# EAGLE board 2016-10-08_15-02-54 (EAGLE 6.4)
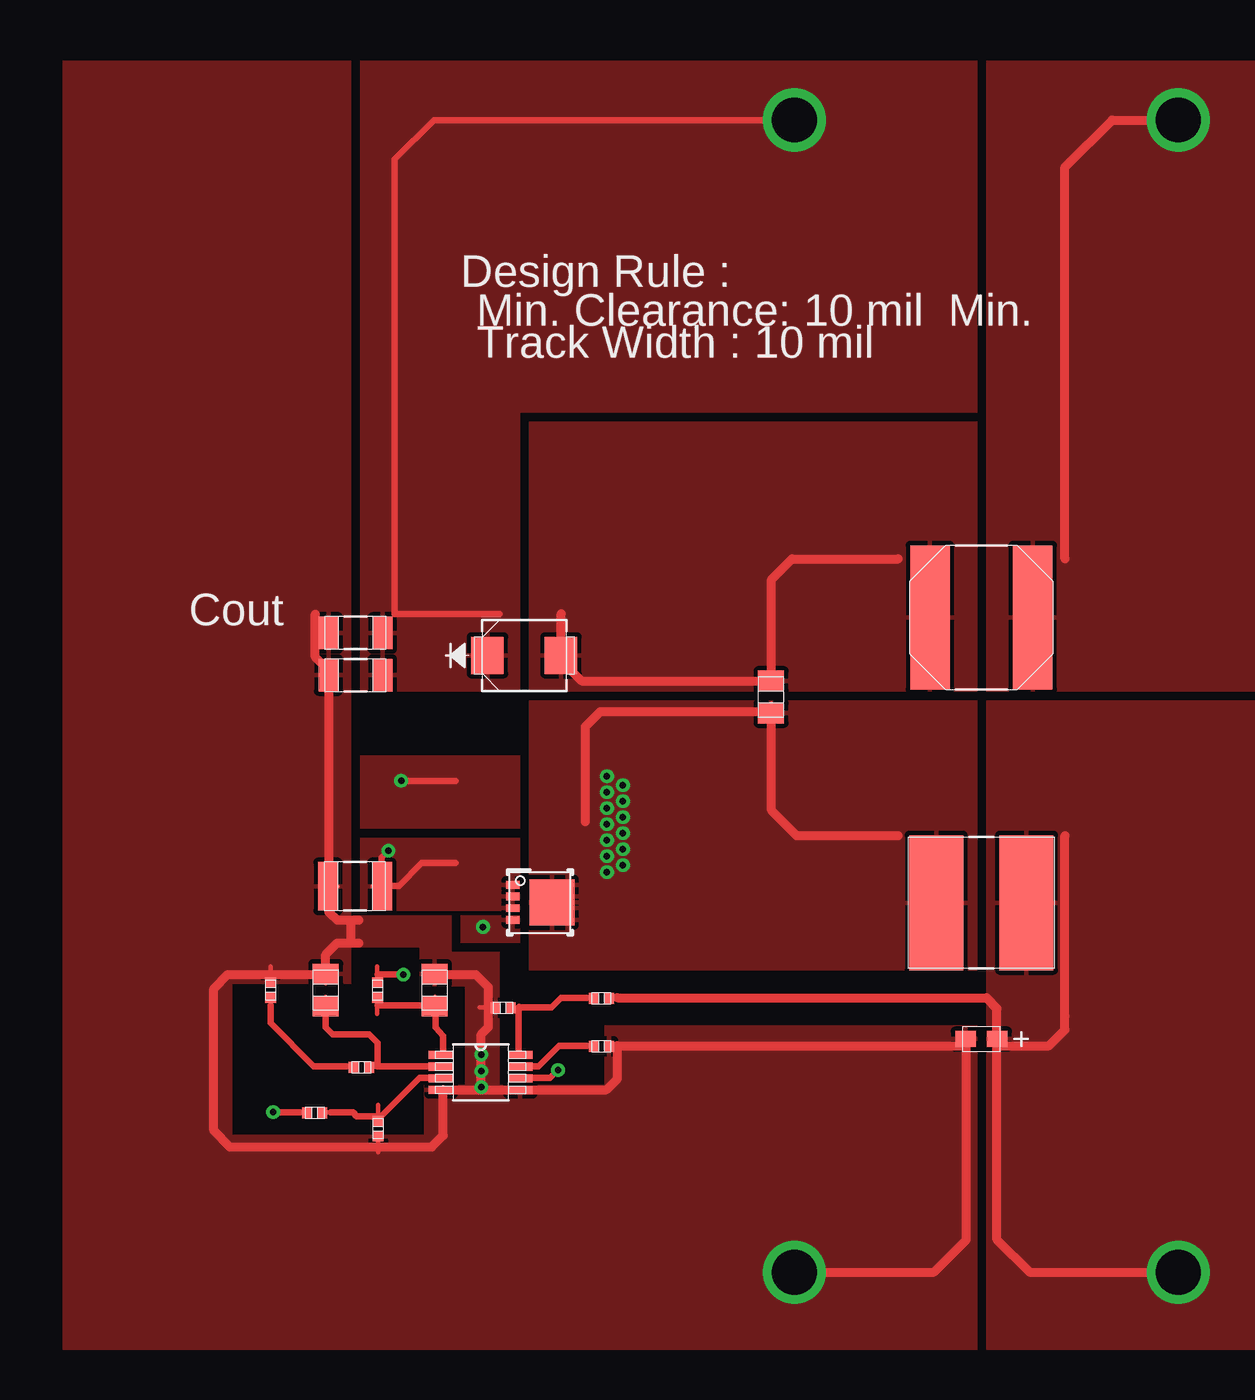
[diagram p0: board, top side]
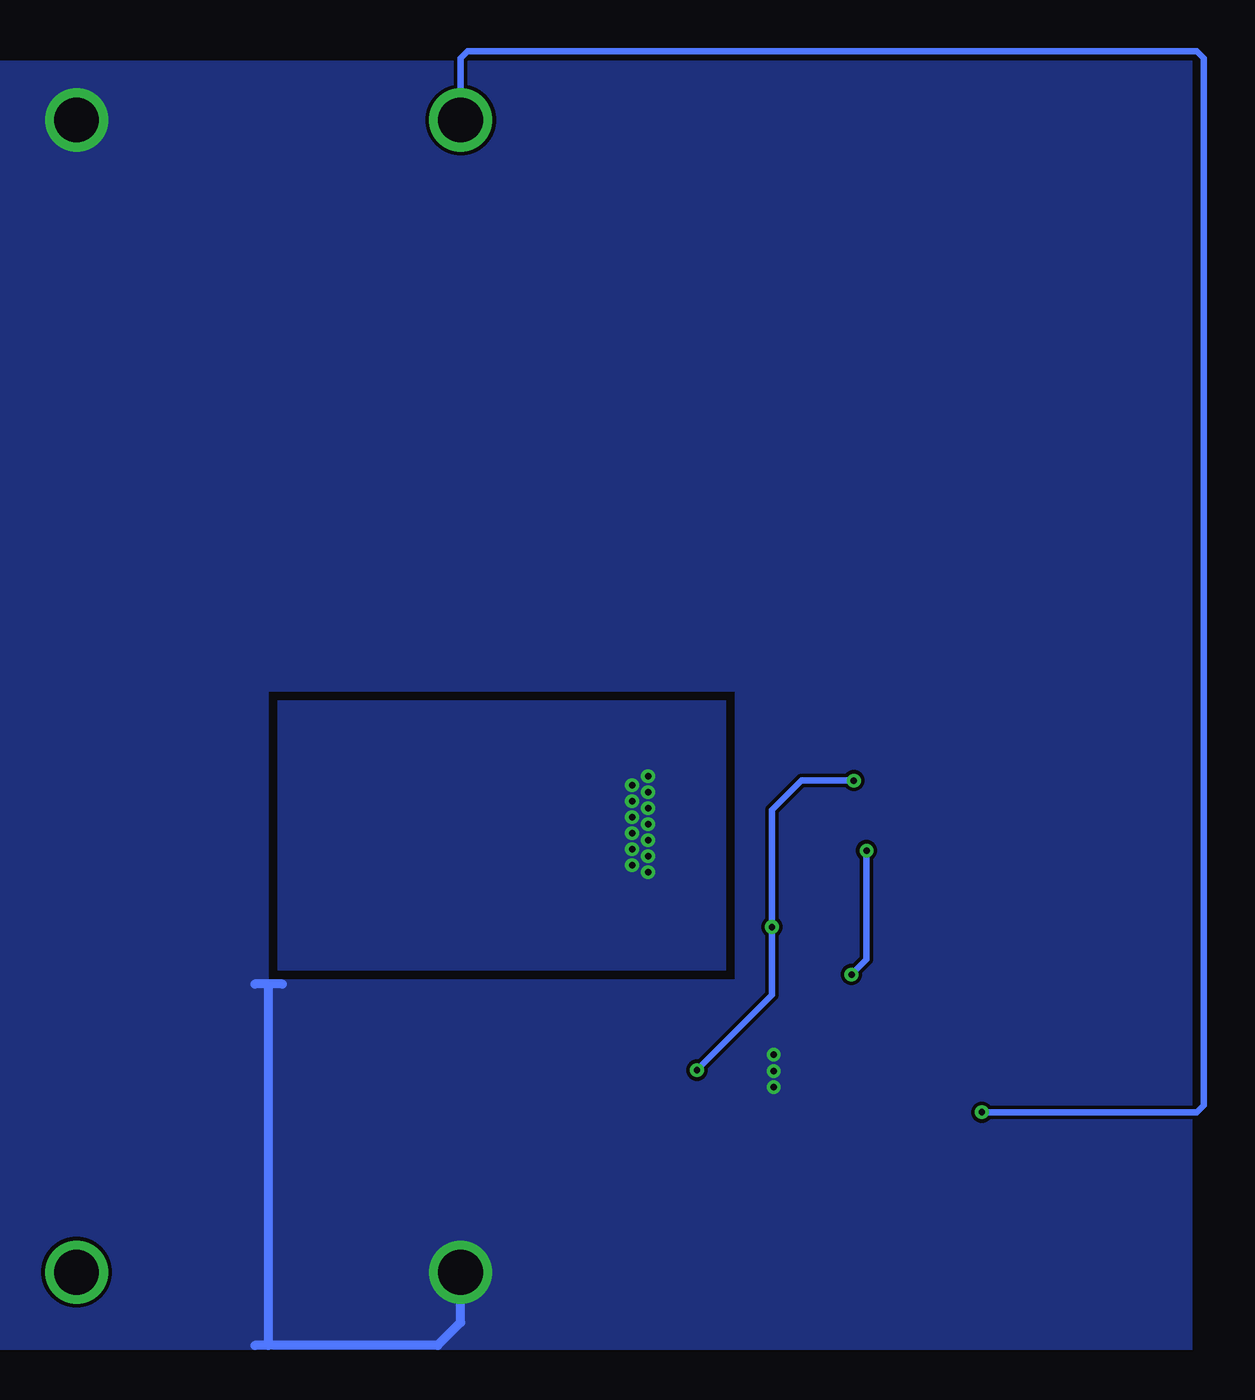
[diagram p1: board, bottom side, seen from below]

No outline drawn. Coordinates in mm, seen from the top.
Copper layers ((1*2)+(15*16)): TOP / INTERNAL1 / layer 15 / BOTTOM

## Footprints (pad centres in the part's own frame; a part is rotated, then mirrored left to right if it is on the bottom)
0402 = smd 0.559 x 0.61: 1 -0.419,0; 2 0.419,0
0805 = smd 1.118 x 1.448: 1 -0.902,0; 2 0.902,0
CAPSMT_6_S09 = smd 1.143 x 0.889: 1 -0.876,0; 2 0.876,0
1206_190 = smd 1.118 x 1.803: 1 -1.499,0; 2 1.499,0
SMB = smd 1.803 x 2.057: 1 -2.045,0; 2 2.045,0
TP-1502 = drill 0.813 round: 1 0,0
IND_NPI75C = smd 2.997 x 7.493: 1 -2.502,0; 2 2.502,0
SRN8040 = smd 2.2 x 8: 1 -2.85,0; 2 2.85,0
DQG0008A = smd 0.75 x 0.44: 1 -1.525,0.975; 2 -1.525,0.325; 3 -1.525,-0.325; 4 -1.525,-0.975; 5 1.525,-0.975; 6 1.525,-0.325; 7 1.525,0.325; 8 1.525,0.975 | smd 2.5 x 2.55: 9 0.65,0
1210 = smd 1.118 x 2.692: 1 -1.499,0; 2 1.499,0
MUA08A = smd 1.372 x 0.457: 1 -2.197,0.975; 2 -2.197,0.325; 3 -2.197,-0.325; 4 -2.197,-0.975; 5 2.197,-0.975; 6 2.197,-0.325; 7 2.197,0.325; 8 2.197,0.975

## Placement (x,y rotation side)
Cbp  [0402]  51.13,45.67 180 top
Ccomp  [0402]  38.2,46.66 90 top
Ccomp2  [0805]  41.27,46.66 90 top
Cin  [CAPSMT_6_S09]  77.7,43.94 180 top
Cout_1  [1206_190]  42.93,64.16 180 top
Cout_2  [1206_190]  42.93,66.5 180 top
Cramp  [0805]  47.32,46.66 90 top
Csep  [0805]  66.01,62.94 270 top
D1  [SMB]  52.3,65.25 0 top
GND  [TP-1502]  67.28,30.96 270 top
GND1  [TP-1502]  88.65,95 270 top
Lin  [IND_NPI75C]  77.7,51.51 0 top
Lout  [SRN8040]  77.7,67.36 0 top
M1  [DQG0008A]  53.19,51.54 0 top
Rbp  [0402]  56.59,46.2 180 top
Rcomp  [0402]  43.26,42.37 180 top
Rfadj  [0402]  56.59,43.54 180 top
Rfb1  [0402]  44.2,38.96 270 top
Rfb2  [0402]  40.67,39.85 0 top
Rramp  [0402]  44.15,46.66 90 top
Rsense  [1210]  42.9,52.43 180 top
U1  [MUA08A]  49.89,42.09 0 top
VIN  [TP-1502]  88.65,30.96 270 top
VOUT  [TP-1502]  67.28,95 270 top

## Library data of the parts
Cbp = ultra-librarian; RefDes: Cbp; Type: GRM155R61A104KA01D
Ccomp = ultra-librarian; RefDes: Ccomp; Type: GRM155R61A823KA01D
Ccomp2 = ultra-librarian; RefDes: Ccomp2; Type: GRM2195C1H512JA01D
Cin = ultra-librarian; RefDes: Cin; Type: 10TPU4R7MSI
Cout_1 Cout_2 = ultra-librarian
Cramp = ultra-librarian; RefDes: Cramp; Type: CL21C122JBFNNWE
Csep = ultra-librarian; RefDes: Csep; Type: GRM21BR71A225KA01L
D1 = ultra-librarian; RefDes: D1; Type: B220-13-F
GND = ultra-librarian; RefDes: GND; Type: TP-1502
GND1 = ultra-librarian; RefDes: GND1; Type: TP-1502
Lin = ultra-librarian; RefDes: Lin; Type: NPI75C120MTRF
Lout = ultra-librarian; RefDes: Lout; Type: SRN8040-330M
M1 = ultra-librarian; RefDes: M1; Type: CSD17308Q3
Rbp = ultra-librarian; RefDes: Rbp; Type: CRCW040220R0FKED
Rcomp = ultra-librarian; RefDes: Rcomp; Type: CRCW04021K18FKED
Rfadj = ultra-librarian; RefDes: Rfadj; Type: CRCW040269K8FKED
Rfb1 = ultra-librarian; RefDes: Rfb1; Type: CRCW040210K0FKED
Rfb2 = ultra-librarian; RefDes: Rfb2; Type: CRCW040216K2FKED
Rramp = ultra-librarian; RefDes: Rramp; Type: CRCW0402100RFKED
Rsense = ultra-librarian; RefDes: Rsense; Type: ERJ-L14KF33MU
U1 = ultra-librarian; RefDes: U1; Type: LM3488MMX/NOPB
VIN = ultra-librarian; RefDes: VIN; Type: TP-1502
VOUT = ultra-librarian; RefDes: VOUT; Type: TP-1502

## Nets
0: Cbp.2 Ccomp2.2 Ccomp.2 Cin.2 Cout_1.2 Cout_2.2 Cramp.2 GND1.1 GND.1 Lout.2 Rfadj.1 Rfb1.2 Rsense.2 U1.4 U1.5
2: Cout_1.1 Cout_2.1 D1.1 Rfb2.1 VOUT.1
3: Cin.1 Lin.2 Rbp.1 VIN.1
4: Ccomp2.1 Rcomp.1 U1.2
5: Csep.1 D1.2 Lout.1
7: Cbp.1 Rbp.2 U1.8
8: Rfb1.1 Rfb2.2 U1.3
9: M1.1 M1.2 M1.3 Rramp.2 Rsense.1
10: Csep.2 Lin.1 M1.5 M1.6 M1.7 M1.8 M1.9
12: Cramp.1 Rramp.1 U1.1
13: Ccomp.1 Rcomp.2
20: M1.4 U1.6
21: Rfadj.2 U1.7

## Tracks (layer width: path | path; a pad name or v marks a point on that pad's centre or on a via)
0  (via drill 0.36 pad 0.64, 2.49 pad 3.48)
  TOP 0.254: 49.84,45.71 50.77,45.71 | 41.26,47.04 41.26,47.98 | 38.21,47.04 38.21,47.98 | 47.36,47.04 47.36,47.98 | 57,43.55 57.94,43.55 | 44.18,37.64 44.18,38.58 | 41,52.43 41.94,52.43
  TOP 0.508: GND1.1 84.96,95 82.35,92.38 82.35,70.61 | v67.31,30.99 75.06,30.99 76.86,32.79 76.86,43.56 57.48,43.56 57.48,41.73 56.87,41.12 47.8,41.12 47.8,38.58 47.17,37.95 35.94,37.95 35.05,38.86 35.05,46.74 35.84,47.52 38.23,47.52 41.27,47.52 41.27,48.64 41.91,49.28 42.67,49.28 | 47.37,47.52 49.61,47.52 50.32,46.81 50.32,45.72 50.32,44.6 49.91,44.2 v49.91,43.08 v49.91,42.16 v49.91,41.27 | 42.67,50.55 43.1,50.55 | 42.67,50.55 41.91,50.55 41.45,50.98 41.45,52.45 41.45,64.41 40.69,65.18 40.69,67.54 | 42.67,49.28 43.1,49.28 | 42.67,49.28 42.67,50.55
  BOTTOM 0.508: 77.98,26.92 68.58,26.92 67.31,28.19 v67.31,30.99 | 77.98,46.99 78.74,46.99 | 77.98,26.92 78.74,26.92 | 77.22,46.99 77.98,46.99 | 77.98,26.92 77.98,46.99
  other vias: 88.65,95
  pour TOP (rank 5): 77.98,98.3 77.98,63.25 132.84,63.25 132.84,98.3
  pour TOP (rank 5): 77.47,44.7 77.47,26.67 26.67,26.67 26.67,98.3 42.67,98.3 42.67,46.99 36.07,46.99 36.07,38.61 46.74,38.61 46.74,41.4 49.02,41.4 49.02,46.86 46.48,46.86 46.48,49.02 42.8,49.02 42.8,50.8 48.26,50.8 48.26,48.77 50.93,48.77 50.93,41.4 56.77,41.4 56.77,44.7
  pour BOTTOM (rank 6): 77.98,26.67 77.98,63.25 52.07,63.25 52.07,47.24 77.72,47.24 77.72,26.67 26.67,26.67 26.67,98.3 132.84,98.3 132.84,26.67
2  (via drill 0.36 pad 0.64, 2.49 pad 3.48)
  TOP 0.254: 39.37,39.87 40.31,39.87
  TOP 0.356: v38.35,39.88 39.85,39.88 | v67.31,95 47.3,95 45.11,92.81 45.11,67.54 45.14,67.56 50.93,67.56
  BOTTOM 0.356: v38.35,39.88 26.42,39.88 26.04,40.26 26.04,98.42 26.42,98.81 66.93,98.81 67.31,98.42 v67.31,95
  pour TOP (rank 3): 77.47,98.3 77.47,78.74 52.07,78.74 52.07,63.25 43.18,63.25 43.18,98.3
3  (via drill 2.49 pad 3.48)
  TOP 0.254: 57,46.22 57.94,46.22
  TOP 0.508: v88.65,30.99 80.39,30.99 78.56,32.79 78.56,43.56 | 57.48,46.23 77.98,46.23 78.56,45.62 78.56,43.56 | 78.56,43.56 81.46,43.56 82.35,44.45 | 82.35,44.45 82.35,45.21 | 82.35,44.45 82.35,55.24
  pour TOP (rank 4): 77.98,62.74 132.84,62.74 132.84,26.67 77.98,26.67
4
  TOP 0.254: 41.26,45.34 41.26,46.28 | 43.66,42.41 44.6,42.41
  TOP 0.356: 47.8,42.42 44.15,42.42 44.15,43.71 43.69,44.2 41.66,44.2 41.27,44.58 41.27,45.82
5
  TOP 0.254: 66.03,63.35 66.03,64.29
  TOP 0.508: 73.08,70.61 67.18,70.61 66.04,69.47 66.04,63.83 55.5,63.83 54.36,64.97 54.36,67.56
  pour TOP (rank 3): 52.58,63.25 77.47,63.25 77.47,78.23 52.58,78.23
7
  TOP 0.254: 51.54,45.71 52.48,45.71 | 55.3,46.22 56.24,46.22
  TOP 0.356: 51.99,43.08 51.99,45.7 | 51.99,45.7 52.02,45.72 | 51.99,45.7 53.82,45.7 54.36,46.23 55.78,46.23
8
  TOP 0.254: 44.18,39.34 44.18,40.28 | 41.07,39.87 42.01,39.87
  TOP 0.356: 41.55,39.88 42.8,39.88 43,39.65 44.35,39.65 46.48,41.78 47.8,41.78
9  (via drill 0.36 pad 0.64)
  TOP 0.254: 44.13,47.04 44.13,47.98 | 43.89,52.43 44.83,52.43
  TOP 0.356: v44.76,54.41 44.37,54.03 44.37,52.45 44.76,52.45 45.34,52.45 46.61,53.72 48.49,53.72 | 44.15,47.52 v45.59,47.52 | v45.59,47.52
  BOTTOM 0.356: v44.76,54.41 44.76,48.36 v45.59,47.52
  pour TOP: 43.18,55.12 52.07,55.12 52.07,51.05 43.18,51.05
10  (via drill 0.36 pad 0.64)
  TOP 0.254: 66.03,61.65 66.03,62.59
  TOP 0.508: 73.08,55.24 67.44,55.24 66.04,56.64 66.04,62.13 56.54,62.13 55.7,61.29 55.7,56.01
  other vias: 57.78,58.04 57.78,57.15 57.78,55.37 57.78,56.26 57.78,54.48 57.78,53.59 56.9,53.21 56.9,54.1 56.9,54.99 56.9,55.88 56.9,56.77 56.9,57.66 56.9,58.55
  pour TOP (rank 2): 52.58,62.74 52.58,47.75 77.47,47.75 77.47,62.74
  pour BOTTOM (rank 4): 52.58,47.75 77.47,47.75 77.47,62.74 52.58,62.74
12
  TOP 0.254: 47.36,45.34 47.36,46.28 | 44.13,45.34 44.13,46.28
  TOP 0.356: 47.8,43.08 47.8,44.12 47.37,44.58 47.37,45.82 44.15,45.82 | 44.15,45.82
13
  TOP 0.254: 38.21,45.34 38.21,46.28 | 41.96,42.41 42.9,42.41
  TOP 0.356: 42.44,42.42 40.62,42.42 38.23,44.83 38.23,45.82
20  (via drill 0.36 pad 0.64)
  TOP 0.356: 51.99,41.78 53.75,41.78 v54.18,42.22 | 48.49,58.27 45.47,58.27 v45.47,58.29
  BOTTOM 0.356: v54.18,42.22 50.01,46.38 v50.01,50.16 50.01,56.67 48.39,58.29 v45.47,58.29
  pour TOP: 43.18,59.69 43.18,55.63 52.07,55.63 52.07,59.69
  pour TOP (rank 2): 52.07,50.8 52.07,49.28 48.77,49.28 48.77,50.8
21
  TOP 0.254: 55.3,43.55 56.24,43.55
  TOP 0.356: 51.99,42.42 53.09,42.42 54.23,43.56 55.78,43.56

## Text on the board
ASSYNOTES: Design Rule : | Min. Clearance: 10 mil Min. | Track Width : 10 mil | Cout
